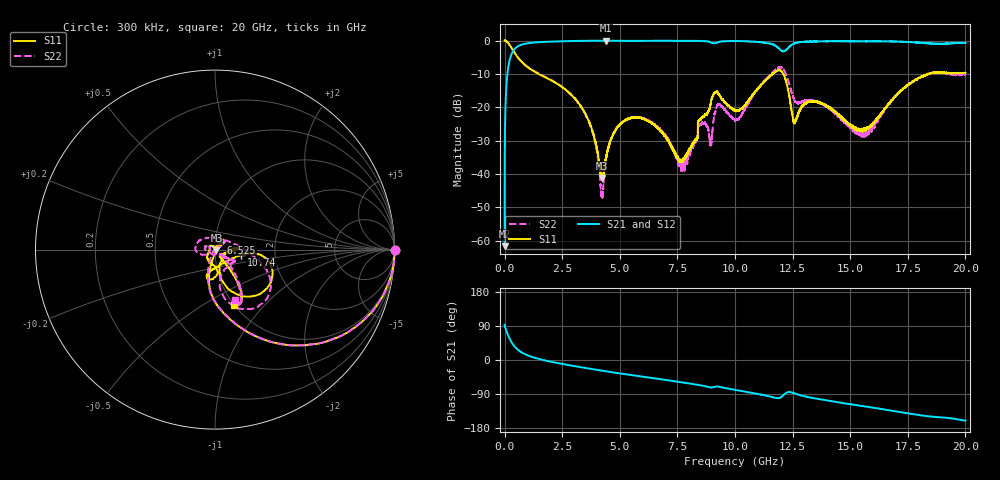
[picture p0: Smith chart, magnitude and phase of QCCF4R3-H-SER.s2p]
!QCCF4R3
!Johanson Technology Inc.
!www.johansontechnology.com
!Test Board Conditions:
!Substrate Type  RO4350B
!Substrate Thickness  10 mil
!Substrate Dk  3.66
!TL Type: GCPW
!TL Trace Width  21 mil
!TL Gap  20 mil
!Electrode orientation  Horizontal
!DUT TOPOLOGY	SERIES
!Mounting Pad LxW  16x21 mil
# MHz S  dB  R 50
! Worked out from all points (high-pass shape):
!   20001 points, 300 kHz to 20 GHz, reference 50 ohm
!   highest |S21| = -0.03 dB at 4.398 GHz (marker M1); lowest = -61.6 dB at 300 kHz (marker M2)
!   |S21| within 3 dB of the highest: 378.4 MHz to 12.01 GHz (11.64 GHz wide, 188 % of centre); 12.18 GHz to end of sweep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
!   lowest |S11| = -41.2 dB at 4.241 GHz (marker M3), VSWR 1.02, Z = 50.8 - j0.306 ohm
!   |S11| at or under -10 dB: 1.477 GHz to 11.63 GHz (10.15 GHz wide, 155 % of centre); 12.09 GHz to 18.42 GHz (6.323 GHz wide, 41.4 % of centre); 18.41819 GHz to 18.42002 GHz (1.839 MHz wide, 0.00998 % of centre)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
!   |S22| runs from -47.2 to 0.0 dB; largest |S21 - S12| = 0.028
!   S11 on the Smith chart (normalised r, x): 300 kHz: open; 6.525 GHz: 1.07, +0.09; 10.74 GHz: 1.34, -0.09; 20 GHz: 1.00, -0.69
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0.3  0.03 -0.2  -61.61 93.1  -61.21 90.2  0.03 -0.0
118.298  -0.42 -19.4  -10.23 70.4  -10.25 70.5  -0.43 -19.5
365.295  -2.93 -48.5  -3.18 41.0  -3.16 41.1  -2.95 -48.5
1139.283  -8.63 -80.8  -0.68 9.2  -0.67 9.1  -8.55 -80.1
3334.25  -19.97 -104.7  -0.09 -19.3  -0.08 -19.2  -20.04 -111.0
3858.242  -28.06 -100.7  -0.06 -24.5  -0.05 -24.5  -28.41 -121.2
4241.236  -41.18 -20.2  -0.04 -28.3  -0.04 -28.2  -46.75 127.0
4398.234  -35.30 33.9  -0.03 -29.8  -0.04 -29.8  -36.13 71.1
5178.222  -24.11 54.5  -0.08 -36.9  -0.06 -36.9  -24.10 50.1
6525.202  -25.51 48.4  -0.08 -48.6  -0.09 -48.6  -25.22 36.7
6667.2  -26.35 47.7  -0.07 -49.9  -0.08 -49.9  -25.99 35.3
7729.184  -35.91 96.4  -0.08 -59.3  -0.07 -59.3  -37.28 -37.0
8950.166  -18.70 -84.9  -0.58 -72.5  -0.55 -72.6  -31.40 177.4
9130.163  -15.62 -95.3  -0.78 -70.8  -0.77 -70.6  -21.69 -160.6
10000.15  -20.82 -69.2  -0.14 -78.8  -0.16 -78.6  -23.85 87.9
10735.14  -16.51 -12.0  -0.31 -86.7  -0.25 -86.7  -16.89 5.5
11961.12  -8.91 -40.0  -2.70 -99.4  -2.80 -99.8  -8.01 -48.4
12579.11  -24.78 -36.3  -0.85 -88.1  -0.87 -88.1  -17.90 -67.4
13334.1  -18.28 3.4  -0.31 -99.6  -0.32 -99.7  -17.99 -30.7
15585.07  -26.76 -51.7  -0.23 -121.8  -0.17 -122.1  -27.77 -43.8
16667.05  -19.03 -53.2  -0.23 -132.5  -0.21 -133.0  -18.82 -44.3
20000  -9.71 -70.9  -0.70 -160.0  -0.55 -158.8  -10.33 -68.5
